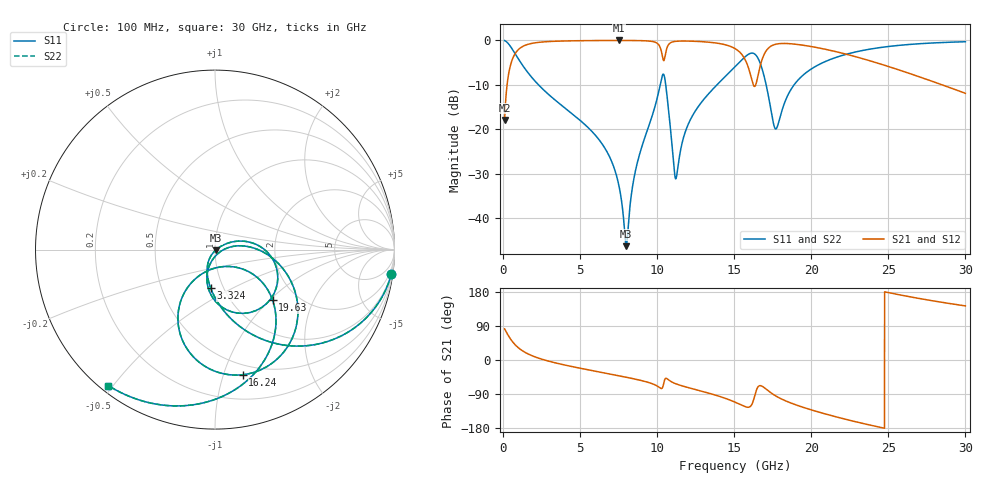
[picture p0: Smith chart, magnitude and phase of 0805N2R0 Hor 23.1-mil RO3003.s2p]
# GHz S MA R 50
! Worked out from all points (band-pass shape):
!   3201 points, 100 MHz to 30 GHz, reference 50 ohm
!   highest |S21| = -0.04 dB at 7.51 GHz (marker M1); lowest = -17.9 dB at 100 MHz (marker M2)
!   |S21| within 3 dB of the highest: 776.4 MHz to 10.31 GHz (9.531 GHz wide, 172 % of centre); 16.96 GHz to 22.16 GHz (5.205 GHz wide, 26.6 % of centre)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
!   lowest |S11| = -46.3 dB at 7.995 GHz (marker M3), VSWR 1.01, Z = 50.3 - j0.348 ohm
!   |S11| at or under -10 dB: 2.292 GHz to 10.19 GHz (7.903 GHz wide, 127 % of centre); 10.55 GHz to 13.89 GHz (3.333 GHz wide, 27.3 % of centre); 17.07 GHz to 18.89 GHz (1.821 GHz wide, 10.1 % of centre)
!   |S22| runs from -46.3 to -0.1 dB; largest |S21 - S12| = 0
!   S11 on the Smith chart (normalised r, x): 100 MHz: 1, -14; 3.324 GHz: 0.87, -0.39; 16.24 GHz: 0.41, -1.16; 19.63 GHz: 1.51, -1.04; 30 GHz: 0.02, -0.49
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0.1  0.9919 -7.9  0.1267 82.1  0.1267 82.1  0.9919 -7.9
0.4176875  0.8819 -30.5  0.4709 59.4  0.4709 59.4  0.8819 -30.5
0.8568438  0.6731 -52.6  0.7387 37.3  0.7387 37.3  0.6731 -52.6
1.7445  0.4048 -76.1  0.9129 13.7  0.9129 13.7  0.4048 -76.1
3.323594  0.2163 -96.3  0.9741 -6.9  0.9741 -6.9  0.2163 -96.3
5.089563  0.1218 -111.1  0.9896 -22.4  0.9896 -22.4  0.1218 -111.1
6.668656  0.05865 -121.4  0.9945 -34.9  0.9945 -34.9  0.05865 -121.4
7.509594  0.0235 -121.2  0.9952 -41.5  0.9952 -41.5  0.0235 -121.2
7.995469  0.004825 -45.8  0.9949 -45.5  0.9949 -45.5  0.004825 -45.8
8.630844  0.03657 29.2  0.9928 -51.0  0.9928 -51.0  0.03657 29.2
10.06978  0.2508 4.1  0.9034 -70.5  0.9034 -70.5  0.2508 4.1
10.49025  0.3756 -70.4  0.6366 -51.8  0.6366 -51.8  0.3756 -70.4
11.22841  0.02796 -40.4  0.9737 -63.1  0.9737 -63.1  0.02796 -40.4
12.28425  0.141 8.7  0.9762 -75.8  0.9762 -75.8  0.141 8.7
15.05  0.5043 -27.8  0.8071 -111.2  0.8071 -111.2  0.5043 -27.8
16.23666  0.714 -77.5  0.3155 -107.6  0.3155 -107.6  0.714 -77.5
16.82531  0.4654 -116.1  0.6204 -69.6  0.6204 -69.6  0.4654 -116.1
17.68494  0.1005 -80.5  0.9017 -94.6  0.9017 -94.6  0.1005 -80.5
19.62844  0.4276 -41.3  0.8713 -126.9  0.8713 -126.9  0.4276 -41.3
20.03956  0.4803 -45.6  0.8477 -132.1  0.8477 -132.1  0.4803 -45.6
25.01978  0.8518 -93.4  0.506 177.7  0.506 177.7  0.8518 -93.4
30  0.9628 -128.1  0.2531 142.8  0.2531 142.8  0.9628 -128.1
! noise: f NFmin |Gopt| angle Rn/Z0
0.1  0.001027  0.9423  1.426  0.003982
3.417  0.006537  0.7134  20.61  0.00436
6.743  0.01172  0.6953  38.88  0.006701
10.06  0.06104  0.9052  56.36  0.1098
13.39  0.03424  0.796  72.76  0.02266
16.7  0.2492  0.9631  88.79  0.7795
20.03  0.05748  0.8272  102.8  0.02762
23.35  0.05771  0.8089  115.5  0.0184
26.67  0.06985  0.8263  127.8  0.01699
30  0.09155  0.8572  139.9  0.01685
